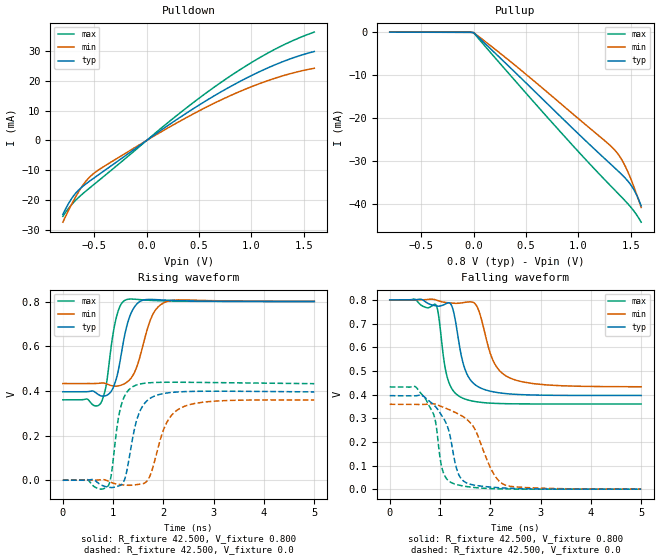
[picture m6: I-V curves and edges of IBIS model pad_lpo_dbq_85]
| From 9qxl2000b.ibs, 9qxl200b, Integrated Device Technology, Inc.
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|   Model pad_lpo_dbq_85
[Model] pad_lpo_dbq_85
Model_type Output
Polarity   Non-Inverting
Vmeas =  0.200V
Cref =  0.0F
Rref =  42.500
Vref =  0.350V
C_comp   1.000fF   1.000fF   1.000fF
[Temperature Range]   65.000   0.125k   -10.000
[Voltage Range]   0.800V   0.800V   0.800V
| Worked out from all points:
|   slope of the pulldown table from 0 to 0.12 V, typ, clamps not added: 40.1 ohm
|   slope of the pullup table from 0 to 0.12 V, typ, clamps not added: 43.1 ohm
|   rising waveform, R_fixture 42.500, V_fixture 0.800: 20-80 % time 221ps typ, 290ps min, 169ps max; typ from 0.396 V to 0.801 V
|   rising waveform, R_fixture 42.500, V_fixture 0.0: 20-80 % time 245ps typ, 341ps min, 176ps max; typ from 0 V to 0.396 V
|   falling waveform, R_fixture 42.500, V_fixture 0.800: 20-80 % time 260ps typ, 351ps min, 197ps max; typ from 0.801 V to 0.396 V
|   falling waveform, R_fixture 42.500, V_fixture 0.0: 20-80 % time 323ps typ, 476ps min, 242ps max; typ from 0.396 V to 0 V
[Pulldown]
|Voltage   I(typ)   I(min)   I(max)
-800mV    -24.75mA   -27.34mA   -25.37mA
-750mV    -21.35mA   -23.69mA   -22.9mA
-700mV    -18.62mA   -20.28mA   -20.82mA
-625mV    -15.8mA    -15.79mA   -18.27mA
-575mV    -14.4mA    -13.41mA   -16.78mA
-500mV    -12.49mA   -10.9mA    -14.63mA
-350mV    -8.768mA   -7.455mA   -10.32mA
275mV     6.702mA    5.611mA    7.986mA
750mV     17.04mA    14.2mA     20.38mA
1.2V      24.91mA    20.51mA    30.03mA
1.4V      27.63mA    22.59mA    33.44mA
1.6V      29.73mA    24.12mA    36.22mA
[Pullup]
|Voltage   I(typ)   I(min)   I(max)
-800mV    81.83uA    71.29uA    95.64uA
0V        -28.42uA   -27.55uA   -40.13uA
350mV     -8.179mA   -6.716mA   -9.928mA
750mV     -17.67mA   -14.85mA   -20.98mA
1.05V     -24.74mA   -21.07mA   -29.04mA
1.325V    -31.01mA   -26.79mA   -36.11mA
1.4V      -32.73mA   -29.02mA   -37.99mA
1.45V     -33.95mA   -31.23mA   -39.27mA
1.525V    -36.37mA   -35.58mA   -41.39mA
1.55V     -37.5mA    -37.23mA   -42.22mA
1.6V      -40.35mA   -40.74mA   -44.16mA
[Ramp]
| variable   typ   min   max
dV/dt_r   0.237/0.245n   0.215/0.344n   0.259/0.176n
dV/dt_f   0.243/0.260n   0.221/0.350n   0.264/0.199n
R_load = 42.500
[Rising Waveform]
R_fixture= 42.500
V_fixture= 0.800
V_fixture_min= 0.800
V_fixture_max= 0.800
|time   V(typ)   V(min)   V(max)
0s        396.2mV    433.2mV    360.3mV
755ps     378.3mV    435.1mV    345.7mV
863ps     379.5mV    432.3mV    427mV
1.022ns   426.9mV    421.5mV    686.2mV
1.133ns   527.6mV    424.1mV    777.5mV
1.253ns   673.7mV    436.1mV    808mV
1.507ns   796.6mV    532.8mV    809.4mV
1.777ns   809.7mV    737.1mV    805.3mV
2.047ns   806.6mV    798.8mV    803.1mV
5ns       800.7mV    800.9mV    800.9mV
[Rising Waveform]
R_fixture= 42.500
V_fixture= 0.0
V_fixture_min= 0.0
V_fixture_max= 0.0
|time   V(typ)   V(min)   V(max)
0s        16.21uV    123.5uV    12.41uV
893ps     -30.42mV   -2.855mV   -27.45mV
962ps     -32.61mV   -9.781mV   22.94mV
1.162ns   -20.33mV   -20.14mV   336.9mV
1.262ns   31.17mV    -21.98mV   390.7mV
1.442ns   246.9mV    -20.23mV   424.7mV
1.702ns   361.5mV    6.13mV     436.2mV
2.032ns   389.5mV    242.7mV    438.8mV
2.352ns   396.2mV    324.6mV    438.8mV
5ns       395.6mV    359.1mV    432.5mV
[Falling Waveform]
R_fixture= 42.500
V_fixture= 0.800
V_fixture_min= 0.800
V_fixture_max= 0.800
|time   V(typ)   V(min)   V(max)
0s        800.7mV    801mV      800.9mV
918ps     775.4mV    800.5mV    779.4mV
968ps     774.1mV    797mV      739.4mV
1.148ns   787.4mV    788.8mV    470.1mV
1.262ns   757mV      786.7mV    416.4mV
1.462ns   530.5mV    789.1mV    384.2mV
1.728ns   437.3mV    775.3mV    369.6mV
2.048ns   412.2mV    547.6mV    363.4mV
2.367ns   403.2mV    472.6mV    361.3mV
5ns       396.2mV    433.2mV    360.3mV
[Falling Waveform]
R_fixture= 42.500
V_fixture= 0.0
V_fixture_min= 0.0
V_fixture_max= 0.0
|time   V(typ)   V(min)   V(max)
0s        395.6mV    359.1mV    432.5mV
500ps     394.7mV    358.5mV    434.5mV
714ps     385.6mV    358.9mV    381.2mV
902ps     351.1mV    359.8mV    294.8mV
1.063ns   302mV      346.4mV    72.14mV
1.264ns   150.9mV    328.4mV    23.99mV
1.485ns   31.75mV    303.2mV    12.64mV
2.075ns   7.622mV    62.12mV    2.006mV
2.295ns   4.632mV    17.55mV    968uV
5ns       16.21uV    123.7uV    12.41uV
